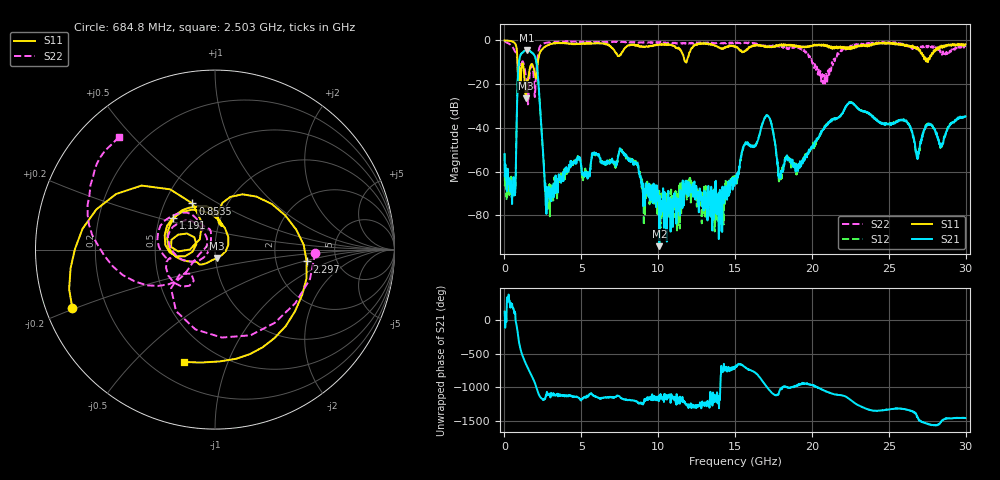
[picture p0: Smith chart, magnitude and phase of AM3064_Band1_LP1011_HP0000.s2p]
# Hz S DB R 50.0
!freq dBS11 angS11 dBS21 angS21 dBS12 angS12 dBS22 angS22
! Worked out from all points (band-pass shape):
!   1600 points, 10 MHz to 29.98 GHz, reference 50 ohm
!   highest |S21| = -4.37 dB at 1.453 GHz (marker M1); lowest = -94.0 dB at 10.08 GHz (marker M2)
!   |S21| within 3 dB of the highest: 1.014 GHz to 1.985 GHz (971.2 MHz wide, 64.8 % of centre)
!   lowest |S11| = -26.4 dB at 1.397 GHz (marker M3), VSWR 1.10, Z = 50.8 - j4.76 ohm
!   |S11| at or under -10 dB: 848.6 MHz to 2.171 GHz (1.322 GHz wide, 87.6 % of centre); 11.80797 GHz to 11.83907 GHz (31.1 MHz wide, 0.263 % of centre)
!   |S22| runs from -29.3 to -0.3 dB; largest |S21 - S12| = 0.0078
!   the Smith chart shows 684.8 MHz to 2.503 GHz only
!   S11 on the Smith chart (normalised r, x): 684.8 MHz: 0.08, -0.20; 853.5 MHz: 0.69, +0.39; 1.191 GHz: 0.59, +0.23; 2.297 GHz: 3.01, -0.54; 2.503 GHz: 0.33, -0.71
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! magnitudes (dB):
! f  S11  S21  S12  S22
! 10 MHz  0.0  -52.0  -51.8  -0.3
! 684.8 MHz  -1.3  -70.7  -66.1  -5.0
! 853.5 MHz  -10.9  -19.9  -19.8  -12.5
! 1.191 GHz  -10.6  -5.5  -5.5  -9.6
! 1.397 GHz  -26.4  -4.4  -4.4  -16.9
! 1.453 GHz  -19.5  -4.4  -4.3  -18.7
! 1.997 GHz  -16.2  -7.6  -7.6  -23.6
! 2.297 GHz  -5.8  -28.6  -28.5  -2.9
! 2.503 GHz  -3.7  -50.5  -50.1  -1.7
! 2.84 GHz  -2.1  -68.7  -68.0  -0.9
! 5.015 GHz  -1.5  -58.6  -59.4  -0.8
! 7.639 GHz  -5.5  -51.1  -50.0  -0.7
! 10 GHz  -2.0  -71.8  -69.8  -1.0
! 10.08 GHz  -2.0  -94.0  -68.8  -1.1
! 15 GHz  -3.0  -65.2  -61.1  -1.4
! 17.05 GHz  -2.9  -34.5  -34.1  -2.9
! 17.95 GHz  -2.4  -62.2  -63.6  -2.5
! 19.99 GHz  -2.7  -49.1  -49.6  -9.4
! 22.47 GHz  -3.2  -28.5  -28.2  -3.2
! 25 GHz  -1.0  -38.1  -38.0  -1.0
! 26.87 GHz  -4.1  -54.3  -53.6  -3.1
! 29.98 GHz  -1.8  -34.7  -35.0  -3.0
